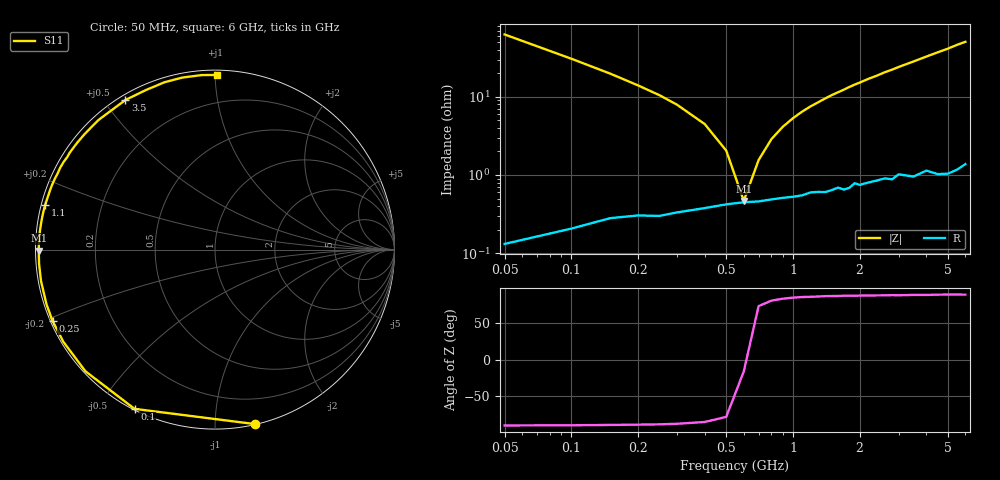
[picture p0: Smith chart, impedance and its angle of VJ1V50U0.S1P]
! Infineon Technologies  Discrete & RF Semiconductors
! BB 914
! Si Tuning Diode in SOT23
! VR = 1.5 V
! S-Parameters:  July  1999
# GHz  S  MA  R  50
!  f  S11
! GHz  MAG  ANG
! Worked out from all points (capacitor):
!   34 points, 50 MHz to 6 GHz, reference 50 ohm
!   read as one part to ground: C = 50.3 pF near 50 MHz
!   lowest |Z| = 466 mohm at 600 MHz (marker M1)
!   series resonance near 608.1 MHz, so ESL is about 1.4 nH
!   S11 on the Smith chart (normalised r, x): 50 MHz: 0.00, -1.26; 100 MHz: 0.00, -0.62; 250 MHz: 0.01, -0.21; 1.1 GHz: 0.01, +0.13; 3.5 GHz: 0.02, +0.57; 6 GHz: 0.03, +1.01
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0.05  0.998 -77.0
0.1  0.994 -116.8
0.15  0.9903 -136.8
0.2  0.9888 -148.7
0.25  0.9886 -156.3
0.3  0.9871 -162.0
0.4  0.9851 -169.8
0.5  0.9833 -175.4
0.6  0.9822 -179.7
0.7  0.9818 176.6
0.8  0.9808 173.5
0.9  0.9799 170.6
1.1  0.9786 165.3
1.4  0.9769 158.4
1.6  0.9741 154.2
1.7  0.9758 152.2
1.9  0.9714 148.0
2.2  0.9716 142.3
2.4  0.9706 138.9
2.6  0.9695 135.1
2.8  0.971 132.0
3  0.9675 128.5
3.5  0.9715 120.9
4  0.9687 113.5
4.5  0.9739 106.8
5  0.9756 100.8
5.5  0.9751 94.4
6  0.9732 89.3
